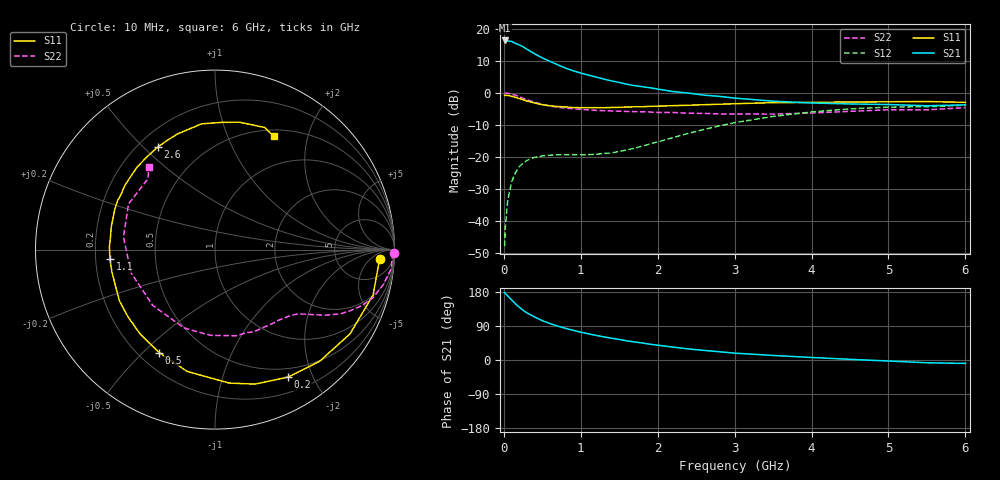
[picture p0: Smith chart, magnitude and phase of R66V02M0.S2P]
! SIEMENS Small Signal Semiconductors
! BFR193
! Si NPN RF Bipolar Junction Transistor in SOT23
! VCE = 6 V  IC = 2 mA
! Common Emitter S-Parameters:  May  1996
# GHz  S  MA  R  50
!  f  S11  S21  S12  S22
! GHz  MAG  ANG  MAG  ANG  MAG  ANG  MAG  ANG
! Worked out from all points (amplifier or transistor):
!   36 points, 10 MHz to 6 GHz, reference 50 ohm
!   highest |S21| = 16.4 dB at 10 MHz (marker M1)
!   |S21| within 3 dB of that: start of sweep to 318 MHz
!   unconditionally stable (mu >= 1): 1.169 GHz to 2.041 GHz
!   at 250 MHz: K = 0.23, MSG = 18.2 dB, |S12| = -22.0 dB
!   at 1.4 GHz: K = 1.11, MAG = 9.2 dB, |S12| = -18.8 dB
!   at 6 GHz: K = 0.99, MSG = 0.1 dB, |S12| = -3.9 dB
!   S11 on the Smith chart (normalised r, x): 10 MHz: 17, -11; 200 MHz: 0.39, -1.66; 500 MHz: 0.28, -0.56; 1.1 GHz: 0.26, -0.04; 2.6 GHz: 0.28, +0.55; 6 GHz: 0.58, +1.48
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0.01  0.9195 -3.2  6.621 178.1  0.004 88.9  0.9981 -1.2
0.02  0.9138 -6.4  6.537 175.5  0.0081 88.7  0.9888 -2.5
0.05  0.9165 -16.0  6.497 169.2  0.0206 80.6  0.9872 -6.2
0.1  0.8867 -32.0  6.402 158.7  0.0402 72.6  0.9569 -11.9
0.15  0.8527 -46.8  5.966 148.2  0.0565 64.8  0.9189 -17.1
0.2  0.8186 -60.2  5.647 139.5  0.0699 58.2  0.8743 -21.0
0.25  0.782 -73.4  5.275 131.2  0.0796 52.3  0.8246 -24.5
0.3  0.7476 -84.0  4.827 124.4  0.088 48.2  0.7833 -27.2
0.4  0.6963 -102.9  4.1 113.6  0.0984 41.2  0.716 -30.7
0.5  0.6527 -118.4  3.534 103.8  0.1035 36.9  0.6629 -33.2
0.6  0.6287 -131.6  3.115 96.1  0.1063 34.3  0.6238 -35.2
0.7  0.6124 -142.5  2.755 89.5  0.1075 33.2  0.5973 -37.0
0.9  0.5902 -160.0  2.221 78.3  0.1084 33.6  0.5647 -40.3
1.1  0.5875 -174.9  1.899 69.1  0.1083 38.1  0.5428 -44.6
1.3  0.5866 173.0  1.646 61.0  0.1125 44.2  0.5268 -49.0
1.6  0.6017 158.2  1.366 50.5  0.1284 54.1  0.5128 -57.0
2.2  0.6321 133.6  1.051 34.0  0.2001 64.3  0.4941 -76.4
2.6  0.6543 119.3  0.924 25.4  0.268 62.7  0.4784 -92.6
3.5  0.7047 96.1  0.743 12.0  0.4287 47.8  0.4659 -138.1
4.5  0.7224 79.3  0.672 1.8  0.5631 26.8  0.5149 172.2
5.5  0.7342 67.9  0.63 -7.3  0.6071 7.3  0.5435 133.4
6  0.7115 62.6  0.65 -9.0  0.6408 2.0  0.5892 128.8
